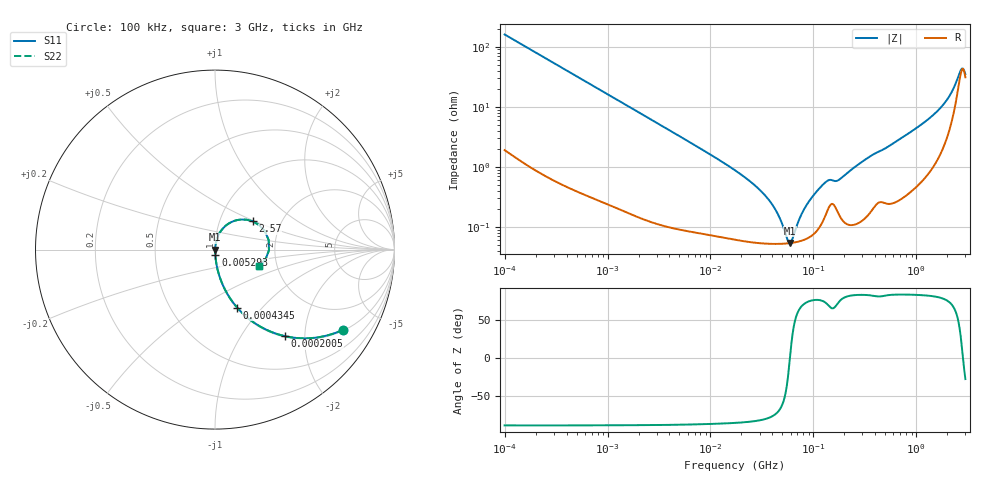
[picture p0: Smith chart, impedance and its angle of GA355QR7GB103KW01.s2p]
!Murata Part Number: GA355QR7GB103KW01
!These Parameters are Measured in Series Mode Connection
!Data Generated on Jun 19, 2026
!  o--ll--o
!Port1  Port2
!  o------o
!Operation Temp=25[degC], DC Bias Voltage=0[V]
!Freq. Start=100[kHz] Stop=3[GHz] 401[Steps]
# Hz S RI R 50
!Freq.(Hz) S11(Real) S11(Imag) S21(Real) S21(Imag) S12(Real) S12(Imag) S22(Real) S22(Imag)
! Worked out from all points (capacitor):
!   401 points, 100 kHz to 3 GHz, reference 50 ohm
!   read as one part in series: C = 9.96 nF near 105.3 kHz
!   lowest |Z| = 54.5 mohm at 59.68 MHz (marker M1)
!   series resonance near 59.18 MHz, so ESL is about 730 pH
!   S11 on the Smith chart (normalised r, x): 100 kHz: 1.04, -3.19; 200.5 kHz: 1.02, -1.60; 434.5 kHz: 1.01, -0.74; 5.293 MHz: 1.00, -0.06; 2.57 GHz: 1.43, +0.49; 3 GHz: 1.62, -0.33
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100000  0.7157 -0.4452  0.2843 0.4452  0.2843 0.4452  0.7157 -0.4452
200542  0.3909 -0.4825  0.6091 0.4825  0.6091 0.4825  0.3909 -0.4825
434500  0.1236 -0.3232  0.8764 0.3232  0.8764 0.3232  0.1236 -0.3232
562235  0.0788 -0.2632  0.9212 0.2632  0.9212 0.2632  0.0788 -0.2632
3161081  0.00374 -0.0513  0.9963 0.0513  0.9963 0.0513  0.00374 -0.0513
5292876  0.00183 -0.0306  0.9982 0.0306  0.9982 0.0306  0.00183 -0.0306
1.77727e7  0.000683 -0.00851  0.9993 0.00851  0.9993 0.00851  0.000683 -0.00851
3.752708e7  0.000534 -0.00268  0.9995 0.00268  0.9995 0.00268  0.000534 -0.00268
4.611977e7  0.000528 -0.00144  0.9995 0.00144  0.9995 0.00144  0.000528 -0.00144
5.667996e7  0.000537 -0.000248  0.9995 0.000248  0.9995 0.000248  0.000537 -0.000248
5.967813e7  0.000542 4.84e-05  0.9995 -4.84e-05  0.9995 -4.84e-05  0.000542 4.84e-05
7.722238e7  0.000598 0.00157  0.9994 -0.00157  0.9994 -0.00157  0.000598 0.00157
9.738194e7  0.000737 0.00308  0.9993 -0.00308  0.9993 -0.00308  0.000737 0.00308
1.361397e8  0.00186 0.00553  0.9981 -0.00553  0.9981 -0.00553  0.00186 0.00553
1.761623e8  0.00168 0.00582  0.9983 -0.00582  0.9983 -0.00582  0.00168 0.00582
3.269943e8  0.00165 0.0135  0.9984 -0.0135  0.9984 -0.0135  0.00165 0.0135
5.475153e8  0.00292 0.0222  0.9971 -0.0222  0.9971 -0.0222  0.00292 0.0222
1.535e9  0.0172 0.076  0.9828 -0.076  0.9828 -0.076  0.0172 0.076
2.145926e9  0.0652 0.1375  0.9348 -0.1375  0.9348 -0.1375  0.0652 0.1375
2.570185e9  0.21 0.1576  0.79 -0.1576  0.79 -0.1576  0.21 0.1576
2.776789e9  0.2993 0.0522  0.7007 -0.0522  0.7007 -0.0522  0.2993 0.0522
3e9  0.2478 -0.0936  0.7522 0.0936  0.7522 0.0936  0.2478 -0.0936
